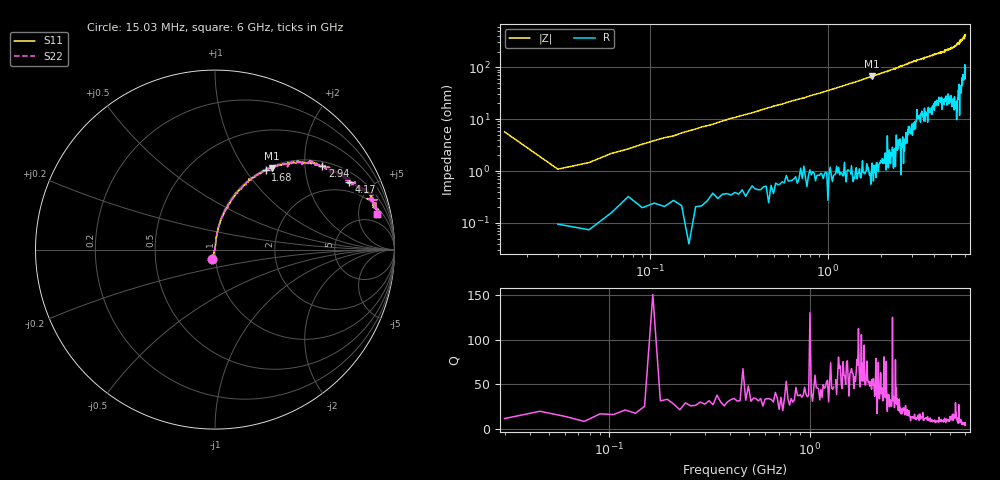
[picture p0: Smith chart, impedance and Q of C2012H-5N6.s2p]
!	Network	Analyzer	HP8753E.07.74:	Oct	30	2002	Serial	No.	JP38451487
!	Hewlett-Packard
!	28	Aug	2009	9:38:54
!	Frequency	S11	S21	S12	S22
#	HZ	S	RI	R	50
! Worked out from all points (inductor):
!   400 points, 15.03 MHz to 6 GHz, reference 50 ohm
!   read as one part in series: L = 5.62 nH near 45.03 MHz
!   highest Q = 71.5 at 1.785 GHz (marker M1), where L = 5.99 nH
!   S11 on the Smith chart (normalised r, x): 15.03 MHz: 0.96, -0.11; 1.68 GHz: 1.02, +1.25; 2.94 GHz: 1.12, +2.46; 4.17 GHz: 1.43, +3.66; 6 GHz: 2.93, +8.15
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1.502992e7  -0.0154 -0.055  1.02 0.055  1.02 0.055  -0.0154 -0.055
3.002985e7  0.00113 0.0108  0.999 -0.0108  0.999 -0.0108  0.00113 0.0108
6.00297e7  0.00205 0.0216  0.998 -0.0216  0.998 -0.0216  0.00205 0.0216
1.050295e8  0.00374 0.0382  0.996 -0.0382  0.996 -0.0382  0.00374 0.0382
1.95029e8  0.00713 0.07  0.993 -0.07  0.993 -0.07  0.00713 0.07
2.850286e8  0.014 0.102  0.986 -0.102  0.986 -0.102  0.014 0.102
5.850271e8  0.0489 0.197  0.951 -0.197  0.951 -0.197  0.0489 0.197
1.020025e9  0.121 0.314  0.879 -0.314  0.879 -0.314  0.121 0.314
1.680022e9  0.283 0.442  0.717 -0.442  0.717 -0.442  0.283 0.442
1.785021e9  0.315 0.454  0.685 -0.454  0.685 -0.454  0.315 0.454
2.01002e9  0.371 0.473  0.629 -0.473  0.629 -0.473  0.371 0.473
2.940015e9  0.598 0.467  0.402 -0.467  0.402 -0.467  0.598 0.467
3.015015e9  0.614 0.468  0.386 -0.468  0.386 -0.468  0.614 0.468
4.00501e9  0.746 0.396  0.254 -0.396  0.254 -0.396  0.746 0.396
4.170009e9  0.748 0.379  0.252 -0.379  0.252 -0.379  0.748 0.379
5.010005e9  0.825 0.339  0.175 -0.339  0.175 -0.339  0.825 0.339
5.565002e9  0.903 0.278  0.097 -0.278  0.097 -0.278  0.903 0.278
5.595002e9  0.862 0.28  0.138 -0.28  0.138 -0.28  0.862 0.28
5.625002e9  0.896 0.251  0.104 -0.251  0.104 -0.251  0.896 0.251
5.925e9  0.889 0.235  0.111 -0.235  0.111 -0.235  0.889 0.235
5.955e9  0.9 0.193  0.1 -0.193  0.1 -0.193  0.9 0.193
6e9  0.904 0.199  0.0959 -0.199  0.0959 -0.199  0.904 0.199
